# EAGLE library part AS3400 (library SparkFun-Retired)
Active noise cancellation chip. Stereo in, stereo out, two microphones. Single alkaline cell power. QFN-24 w/exposed pad. Dead Prototype: IC-10703
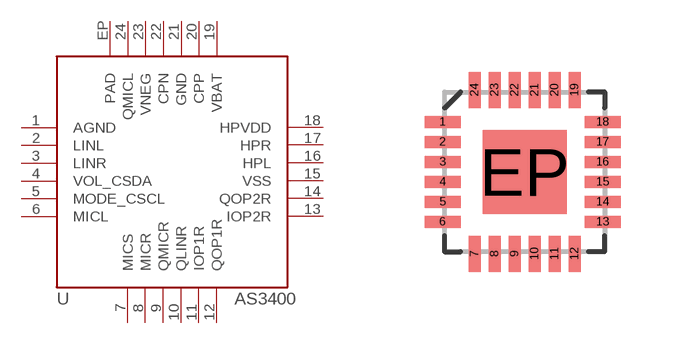
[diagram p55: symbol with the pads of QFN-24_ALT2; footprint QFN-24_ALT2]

Designator prefix U

## AS3400  [QFN-24_ALT2]
1  AGND
2  LINL
3  LINR
4  VOL_CSDA
5  MODE_CSCL
6  MICL
7  MICS
8  MICR
9  QMICR
10  QLINR
11  IOP1R
12  QOP1R
13  IOP2R
14  QOP2R
15  VSS
16  HPL
17  HPR
18  HPVDD
19  VBAT
20  CPP
21  GND
22  CPN
23  VNEG
24  QMICL
EP  PAD

## Footprint QFN-24_ALT2 (pad centres in mm)
24-pin QFN with Exposed Thermal pad Parts that use this package: A6282 Last modified: 8/20/10 ***UNPROVEN***
smd 0.9 x 0.3: 1 -2.05,1.25; 2 -2.05,0.75; 3 -2.05,0.25; 4 -2.05,-0.25; 5 -2.05,-0.75; 6 -2.05,-1.25; 13 1.95,-1.25; 14 1.95,-0.75; 15 1.95,-0.25; 16 1.95,0.25; 17 1.95,0.75; 18 1.95,1.25
smd 0.3 x 0.9: 7 -1.25,-2.05; 8 -0.75,-2.05; 9 -0.25,-2.05; 10 0.25,-2.05; 11 0.75,-2.05; 12 1.25,-2.05; 19 1.25,2.05; 20 0.75,2.05; 21 0.25,2.05; 22 -0.25,2.05; 23 -0.75,2.05; 24 -1.25,2.05
smd 2.1 x 2.1: EP 0,0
